|Texas Instruments Incorporated
|xxxxx
| Marketing part#   Digital Voltage Range   Package-type   #pins
|AMC80AIPW   3.0 to 5.5   TSSOP   24
|AMC80AIPWR   3.0 TO 5.5   TSSOP   24
[IBIS Ver]   4.0
[File name]   amc80.ibs
[File Rev]   1.0
|SimDE V3.0 201101  Build 453
[Date]   08/26/2011
[Source]   Texas Instruments Incorporated.
   Analog-eLab, HPA
   12500 TI Blvd
   Dallas, TX -75243
   For Support e-mail: elab_ibis@list.ti.com
[Notes]   Revision History:
   1.0: 08/26/2011
   - Initial version of the model
   - Initial Model generated from simulations in TISPICED
   - Model names with a trailing _3 contains the model for
   3V (2.7V and 3.3V).
   _ Model names with trailing _5 contains
   the model for 5V (4.75V and 5.25V) operation.
   - Model not matched to measurements
   - C_comp although listed in numerical order of value are
   obtained from varying PVT conditions. For PVT conditions
   for each specific value refer the buffer description under
   respective [Model]. IBIS model user is responsible for using
   appropriate C_comp to simulate for Signal Integrity.
   - Combined Pulldown non-monotonic warnings for SDA_5 and
   SDA_33 typical, minimum, and maximum errors are minimal .
   based on SPICE simulations and accepted.
   - Non-monotonic combined warnings for A0_5, A0_3p3, GPO_5,
   GPO_3p3, INT_5, INT_3p3, GPI_5, GPI_3p3, SDA_5, and
   SDA_3p3 are minor and reflect SPICE transistor simulations
[Disclaimer]
  This model is designed as an aid for customers of Texas Instruments.
  TI and its licensors and suppliers make no warranties, either expressed
  or implied, with respect to this model, including the warranties of
  merchantability or fitness for a particular purpose.  The model is
  provided solely on an "as is" basis.  The entire risk as to its quality
  and performance is with the customer.
[Copyright] (C) Copyright 2011 Texas Instruments Incorporated.
   All rights reserved.
|   AMC80
[Component]   amc80
[Manufacturer] TI
[Package]   | 24 TSSOP - PW package
| variable   typ   min   max
R_pkg   0.177   0.163   0.188
L_pkg   3.366nH  2.841nH  4.068nH
C_pkg   0.530pF  0.433pF  0.650pF
|-------------------------PIN------------------------------------------------
[Pin] signal_name  model_name  R_pin  L_pin C_pin
1   _INT_IN   DIN1  0.16264  4.03972nH  0.64996pF
2   SDA   SDA   0.17685  3.73012nH  0.63154pF
3   SCL   SCL   0.18356  3.37945nH  0.52823pF
4   FAN1   DIN1  0.18796  3.15435nH  0.47111pF
5   FAN2   DIN1  0.18027  2.96398nH  0.46303pF
6   _BTI   DIN1  0.17244  2.84228nH  0.43324pF
7   GPI(C1)   GPI   0.17243  2.84211nH  0.43313pF
8   DGND   GND   0.17967  2.96088nH  0.46295pF
9   V+   POWER 0.18749  3.15347nH  0.47237pF
10  _INT   INT   0.18522  3.39935nH  0.52967pF
11  _GPO   GPO   0.17199  3.69520nH  0.62727pF
12  _NTEST_IN/RESET_IN  DIN1  0.16476  4.06847nH  0.64869pF
13  _RST_OUT/_OS   RST   0.16332  4.05052nH  0.64862pF
14  AGND   GND   0.17180  3.69103nH  0.62832pF
15  CH6   TERM  0.18523  3.39835nH  0.52985pF
16  CH5   TERM  0.18796  3.15774nH  0.47154pF
17  CH4   TERM  0.18027  2.96616nH  0.46313pF
18  CH3   TERM  0.17244  2.84275nH  0.43337pF
19  CH2   TERM  0.17242  2.84098nH  0.43368pF
20  CH1   TERM  0.18026  2.96397nH  0.46337pF
21  CHO   TERM  0.18795  3.15427nH  0.47177pF
22  A0/NTEST_OUT   A0   0.18522  3.39505nH  0.52868pF
23  A1   DIN2  0.17640  3.72891nH  0.62935pF
24  A2   DIN2  0.16480  4.06428nH  0.64933pF
|   Model Selectors
[Model Selector]  DIN1
DIN1_3p3 3.3V digital input
DIN1_5   5V digital input
|NOTES   Model DIN1 split into two Models DIN1_3p3 and DIN1_5
|   to accomodate vast voltage range of 3.0V - 5.5V
|   DIN1_3p3 operates in voltage range of 3 - 3.3 - 3.6
|   DIN1_5 operates in voltage range of 4.5 - 5 - 5.5
|   The max pin frequency for Model DIN1 is 3.4MHz.Also the
|   voltage range and frequency is referenced with datasheet.
[Model Selector]  SDA
SDA_3p3 3.3V digital I/O open drain
SDA_5   5V digital I/O open drain
|NOTES   Model SDA split into two Models SDA_3p3 and SDA_5
|   to accomodate vast voltage range of 3.0V - 5.5V
|   SDA_3p3 operates in voltage range of 3 - 3.3 - 3.6
|   SDA_5 operates in voltage range of 4.5 - 5 - 5.5
|   The max pin frequency for Model SDA is 3.4MHz.Also the
|   voltage range and frequency is referenced with datasheet.
[Model Selector]  SCL
SCL_3p3 3.3V digital input
SCL_5   5V digital input
|NOTES   Model SCL split into two Models SCL_3p3 and SCL_5
|   to accomodate vast voltage range of 3.0V - 5.5V
|   SCL_3p3 operates in voltage range of 3 - 3.3 - 3.6
|   SCL_5 operates in voltage range of 4.5 - 5 - 5.5
|   The max pin frequency for Model SCL is 3.4MHz.Also the
|   voltage range and frequency is referenced with datasheet.
[Model Selector]  GPI
GPI_3p3 3.3V digital I/O open drain
GPI_5   5V digital I/O open drain
|NOTES   Model GPI split into two Models GPI_3p3 and GPI_5
|   to accomodate vast voltage range of 3.0V - 5.5V
|   GPI_3p3 operates in voltage range of 3 - 3.3 - 3.6
|   GPI_5 operates in voltage range of 4.5 - 5 - 5.5
|   The max pin frequency for Model GPI is 3.4MHz.Also the
|   voltage range and frequency is referenced with datasheet.
[Model Selector]  INT
INT_3p3 3.3V digital tri-state
INT_5   5V digital tri-state
|NOTES   Model INT split into two Models INT_3p3 and INT_5
|   to accomodate vast voltage range of 3.0V - 5.5V
|   INT_3p3 operates in voltage range of 3 - 3.3 - 3.6
|   INT_5 operates in voltage range of 4.5 - 5 - 5.5
|   The max pin frequency for Model INT is 3.4MHz.Also the
|   voltage range and frequency is referenced with datasheet.
[Model Selector]  GPO
GPO_3p3 3.3V digital output open drain
GPO_5   5V digital output open drain
|NOTES   Model GPO split into two Models GPO_3p3 and GPO_5
|   to accomodate vast voltage range of 3.0V - 5.5V
|   GPO_3p3 operates in voltage range of 3 - 3.3 - 3.6
|   GPO_5 operates in voltage range of 4.5 - 5 - 5.5
|   The max pin frequency for Model GPO is 3.4MHz.Also the
|   voltage range and frequency is referenced with datasheet.
[Model Selector]  RST
RST_3p3 3.3V digital output open drain
RST_5   5V digital output open drain
|NOTES   Model RST split into two Models RST_3p3 and RST_5
|   to accomodate vast voltage range of 3.0V - 5.5V
|   RST_3p3 operates in voltage range of 3 - 3.3 - 3.6
|   RST_5 operates in voltage range of 4.5 - 5 - 5.5
|   The max pin frequency for Model RST is 3.4MHz.Also the
|   voltage range and frequency is referenced with datasheet.
[Model Selector]  A0
A0_3p3 3.3V digital I/O
A0_5   5V digital I/O
|NOTES   Model A0 split into two Models A0_3p3 and A0_5
|   to accomodate vast voltage range of 3.0V - 5.5V
|   A0_3p3 operates in voltage range of 3 - 3.3 - 3.6
|   A0_5 operates in voltage range of 4.5 - 5 - 5.5
|   The max pin frequency for Model A0 is 3.4MHz.Also the
|   voltage range and frequency is referenced with datasheet.
[Model Selector]  DIN2
DIN2_3p3 3.3V digital input
DIN2_5   5V digital input
|NOTES   Model DIN2 split into two Models DIN2_3p3 and DIN2_5
|   to accomodate vast voltage range of 3.0V - 5.5V
|   DIN2_3p3 operates in voltage range of 3 - 3.3 - 3.6
|   DIN2_5 operates in voltage range of 4.5 - 5 - 5.5
|   The max pin frequency for Model DIN2 is 3.4MHz.Also the
|   voltage range and frequency is referenced with datasheet.
[Model Selector]  TERM
TERM_3p3 3.3V digital input
TERM_5   5V digital input
|   TERM Model
[Model] TERM_3p3
Model_type Terminator
C_comp   1e-20   1e-20   1e-20
| variable   typ   min   max
[Voltage Range]   3.3V   3.0V   3.6V
[POWER Clamp Reference]  3.3V   3.0V   3.6V
[GND Clamp Reference]   0.0V   0.0V   0.0V
|Operating Temperature
[Temperature Range]   27   125   -40
[Model] TERM_5
Model_type Terminator
C_comp   1e-20   1e-20   1e-20
| variable   typ   min   max
[Voltage Range]   5.0V   4.5V   5.5V
[POWER Clamp Reference]  5.0V   4.5V   5.5V
[GND Clamp Reference]   0.0V   0.0V   0.0V
|Operating Temperature
[Temperature Range]   27   125   -40
| Models and submodels in the file (20): DIN1_3p3 (Input), DIN1_5 (Input), SDA_3p3 (I/O_open_drain), SDA_5 (I/O_open_drain), SCL_3p3 (Input), SCL_5 (Input), GPI_3p3 (I/O_open_drain), GPI_5 (I/O_open_drain), INT_3p3 (3-state), INT_5 (3-state), GPO_3p3 (Open_drain), GPO_5 (Open_drain), RST_3p3 (Open_drain), RST_5 (Open_drain), A0_3p3 (I/O), A0_5 (I/O), DIN2_3p3 (Input), DIN2_5 (Input), TERM_3p3 (Terminator), TERM_5 (Terminator)
